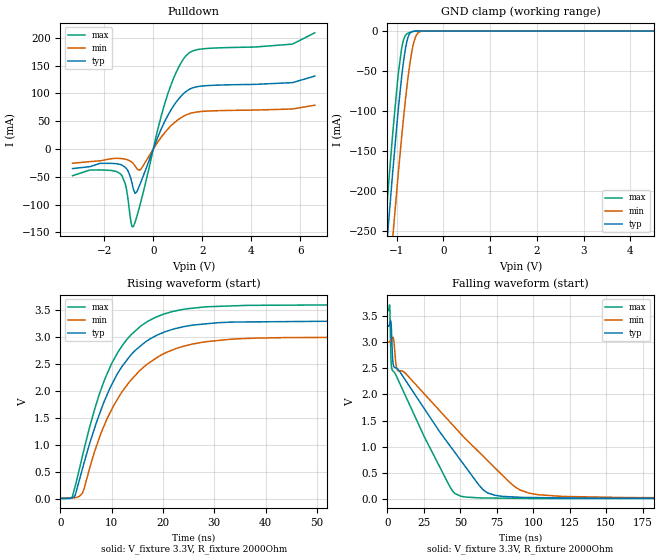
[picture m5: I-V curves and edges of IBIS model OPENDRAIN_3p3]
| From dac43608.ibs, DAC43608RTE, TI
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|   OPENDRAIN_3p3 Model
[Model]   OPENDRAIN_3p3
Model_type   I/O_open_drain
Polarity   Non-Inverting
Enable   Active-Low
Vinl = 0.5
Vinh = 2.4
Vmeas = 1.65
Vref = 3.3
Cref = 2pF
Rref = 2000
|   typ   min   max
C_comp   1.131E-12   1.111E-12   1.158E-12
|  Where Nom  PVT is Nominal Process, 3.3V,   25C
|   Fast PVT is Strong Process,  3.6V,  -40C
|   Slow PVT is Weak Process,   3.0V,  125C
[Voltage Range]   3.3   3   3.6
|Junction Temperature
[Temperature Range]   25   125   -40
[Pullup Reference]   3.3   3   3.6
[Pulldown Reference]   0   0   0
[Power Clamp Reference]   3.3   3   3.6
[GND Clamp Reference]   0   0   0
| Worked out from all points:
|   slope of the pulldown table from 0 to 0.495 V, typ, clamps not added: 9.51 ohm
|   GND clamp passes 1 mA (typ) near -0.68 V on its own axis
|   falling waveform, V_fixture 3.3V, R_fixture 2000Ohm: 20-80 % time 48.4ns typ, 60.7ns min, 31.6ns max; typ from 3.3 V to 0.013 V
|   rising waveform, V_fixture 3.3V, R_fixture 2000Ohm: 20-80 % time 8.88ns typ, 9.89ns min, 8.21ns max; typ from 0.013 V to 3.3 V
[Pulldown]
|   Voltage   I(typ)   I(min)   I(max)
-3.3V     -35.19mA   -25.59mA   -48mA
-1.36V    -27.75mA   -17mA      -44.21mA
-1.142V   -33.05mA   -18.29mA   -63.19mA
-904.2mV  -55.52mA   -22.76mA   -133.4mA
-815.1mV  -72.15mA   -26.34mA   -139.6mA
-745.8mV  -79.88mA   -30.41mA   -131.8mA
-528mV    -61.78mA   -37.27mA   -98.21mA
501.6mV   52.63mA    31.22mA    86.45mA
917.4mV   83.38mA    49.38mA    136.3mA
1.353V    104mA      61.44mA    168.5mA
5.679V    119.4mA    71.98mA    188.7mA
6.6V      131.3mA    78.9mA     209.1mA
[GND Clamp]
|   Voltage   I(typ)   I(min)   I(max)
-3.3V     -1.874A    -1.854A    -1.896A
-1.251V   -296.5mA   -376.3mA   -249.6mA
-1.221V   -274.5mA   -354.8mA   -227.1mA
-1.162V   -231mA     -312.2mA   -182.8mA
-1.082V   -174.8mA   -256.6mA   -126.5mA
-973.5mV  -103mA     -183.1mA   -58.23mA
-894.3mV  -57.67mA   -133mA     -22.06mA
-815.1mV  -23.06mA   -87.31mA   -5.585mA
-735.9mV  -4.714mA   -48.47mA   -2.096mA
-617.1mV  -238.4uA   -10.92mA   -291.6uA
-478.5mV  -7.306uA   -419.8uA   -7.415uA
6.6V      0A         0A         0A
[POWER Clamp]
|   Voltage   I(typ)   I(min)   I(max)
-3.3V     0A         0A         0A
0V        0A         0A         0A
6.6V      0A         0A         0A
[Ramp]
R_load = 2000
|   typ   min   max
dV/dt_r   1.97194/8.86027e-09   1.78763/9.89683e-09   2.15469/8.20902e-09
dV/dt_f   1.97194/4.84455e-08   1.78763/6.06818e-08   2.15469/3.1555e-08
[Falling Waveform]
V_fixture = 3.3V
V_fixture_min = 3V
V_fixture_max = 3.6V
R_fixture = 2000Ohm
C_fixture = 0F
|   Time   V(typ)   V(min)   V(max)
0s        3.3V       3V         3.6V
1.624ns   3.355V     3.005V     3.694V
2.522ns   3.38V      3.046V     2.662V
3.29ns    2.875V     3.08V      2.47V
4.182ns   2.553V     3.066V     2.438V
7.04ns    2.486V     2.457V     2.299V
50.46ns   734.5mV    1.244V     55.6mV
69.33ns   111.9mV    719mV      21.95mV
103.2ns   29.44mV    85.37mV    12.8mV
500ns     13.43mV    20.62mV    8.851mV
[Rising Waveform]
V_fixture = 3.3V
V_fixture_min = 3V
V_fixture_max = 3.6V
R_fixture = 2000Ohm
C_fixture = 0F
|   Time   V(typ)   V(min)   V(max)
0s        13.43mV    20.62mV    8.851mV
2.317ns   27.77mV    23.44mV    49.76mV
2.935ns   91.38mV    30.06mV    263.7mV
4.264ns   554.7mV    111.2mV    791.1mV
7.724ns   1.606V     1.176V     1.987V
9.859ns   2.097V     1.638V     2.489V
12.34ns   2.503V     2.034V     2.886V
19.14ns   3.053V     2.646V     3.394V
27.86ns   3.245V     2.911V     3.56V
500ns     3.3V       3V         3.6V
